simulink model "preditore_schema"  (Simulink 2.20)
settings: Solver=VariableStepDiscrete  StartTime=0.0  StopTime=40.0  RelTol=1e-3  AbsTol=1e-6
libraries: simulink x3

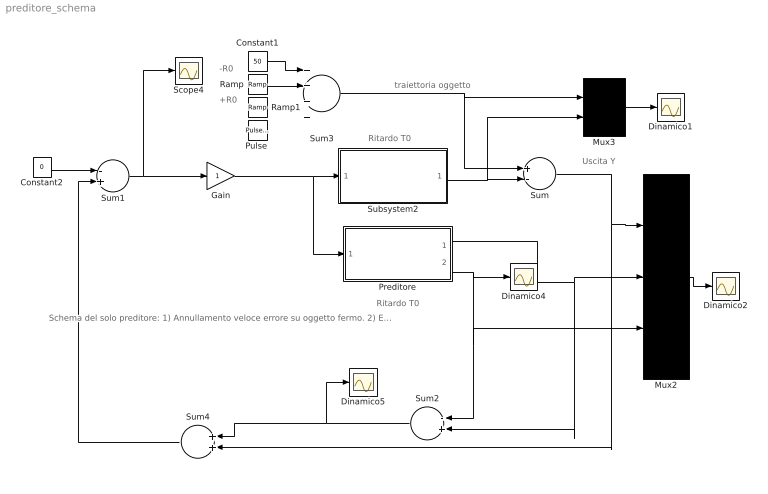
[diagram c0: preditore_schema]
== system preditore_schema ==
  note: traiettoria oggetto
  note: -R0
  note: +R0
  note: Ritardo T0
  note: Ritardo T0
  note: Uscita Y
  note: Schema del solo preditore: 1) Annullamento veloce errore su oggetto fermo. 2) Errore a regime su oggetto in movimento, ma questo sarebbe atteso dato che un proporzionale Kp=1 non e' di per se in grado di annullare l'errore a regime.
  Constant1 : Constant  Value=50
  Constant2 : Constant  Value=0
  Dinamico{1..2,4..5} (4 alike) : Scope
  Gain : Gain  Gain=1
  Mux2 : Mux  Inputs=3
  Mux3 : Mux  Inputs=2
  Preditore : Subsystem  mask(Modello del Puma 260 in Alter Mode){Ts=.260}
      mask prompts: Ts "Tempo di Campionamento Ts della seriale"
      mask help: Questo blocco racchiude il comportamento dinamico del Puma 260 pilotato dalla seriale. La rappresentazione e' a variabili di stato.
      mask init:
      | K=10; % attenuazione del guadagno puma.
      | A=[0,0,0,0,0,0,0,0,0,0;
      | 1,0,0,0,0,0,0,0,0,0;
      | 0,1,0,0,0,0,0,0,0,0;
      | 0,0,1,0,0,0,0,0,0,0;
      | 0,0,0,1,0,0,0,0,0,0;
      | 0,0,0,0,1,0,0,0,0,0;
      | 0,0,0,0,0,1,0,0,0,0;
      | 0,0,0,0,0,0,1,0,0,0;
      | 0,0,0,0,0,0,0,1,0,0;
      | 0,0,0,0,0,0,0,0,1/K,1];
      | B=[1;0;0;0;0;0;0;0;0;0];
      | C=[0,0,0,0,0,0,0,0,0,1;
      | 1/K,1/K,1/K,1/K,1/K,1/K,1/K,1/K,1/K,1];
      | D=[0;0];
  "Pulse " : simulink/Sources/Pulse Generator  period=30  duty=10  amplitude=-50  start=30
  Ramp : simulink/Sources/Ramp  slope=-26  start=10  X0=0
  Ramp1 : simulink/Sources/Ramp  slope=+50  start=25  X0=0
  Scope4 : Scope
  Subsystem2 : Subsystem  mask(Modello del Puma 260 in Alter Mode){Ts=.260}
      mask prompts: Ts "Tempo di Campionamento Ts della seriale"
      mask help: Questo blocco racchiude il comportamento dinamico del Puma 260 pilotato dalla seriale. La rappresentazione e' a variabili di stato.
      mask init:
      | K=10; % attenuazione del guadagno puma.
      | A=[0,0,0,0,0,0,0,0,0,0;
      | 1,0,0,0,0,0,0,0,0,0;
      | 0,1,0,0,0,0,0,0,0,0;
      | 0,0,1,0,0,0,0,0,0,0;
      | 0,0,0,1,0,0,0,0,0,0;
      | 0,0,0,0,1,0,0,0,0,0;
      | 0,0,0,0,0,1,0,0,0,0;
      | 0,0,0,0,0,0,1,0,0,0;
      | 0,0,0,0,0,0,0,1,0,0;
      | 0,0,0,0,0,0,0,0,1/K,1];
      | B=[1;0;0;0;0;0;0;0;0;0];
      | C=[0,0,0,0,0,0,0,0,0,1];
      | D=[0];
  Sum : Sum  Inputs=+-
  Sum1 : Sum  Inputs=-+
  Sum2 : Sum  Orientation=left  Inputs=-+
  Sum3 : Sum  Inputs=++++
  Sum4 : Sum  Orientation=left  Inputs=++
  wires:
  Mux2/1 -> Dinamico2/1
  Subsystem2/1(Out1) -> Sum/2, Mux3/2
  Mux3/1 -> Dinamico1/1
  Constant1/1 -> Sum3/1
  Sum/1 -> Mux2/1, Sum4/2
  Preditore/1(Out1) -> Mux2/2, Sum2/2
  Preditore/2(Out2) -> Dinamico4/1, Sum2/1, Mux2/3
  Sum3/1 -> Mux3/1, Sum/1
  Sum1/1 -> Scope4/1, Gain/1
  Sum4/1 -> Sum1/2
  Constant2/1 -> Sum1/1
  Sum2/1 -> Sum4/1, Dinamico5/1
  Ramp/1 -> Sum3/2
  Gain/1 -> Subsystem2/1(In1), Preditore/1(In1)

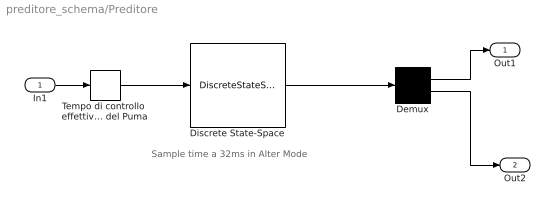
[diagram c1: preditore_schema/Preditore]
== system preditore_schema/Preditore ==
  note: Sample time a 32ms in Alter Mode
  In1 : Inport  Port=1  PortWidth=-1  SampleTime=-1
  Demux : Demux  Outputs=2
  Discrete State-Space : DiscreteStateSpace  A=A  B=B  C=C  D=D  X0=0  SampleTime=.033
  Tempo di controllo  effettivo Ts del Puma : ZeroOrderHold  SampleTime=Ts
  Out1 : Outport  Port=1
  Out2 : Outport  Port=2
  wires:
  In1/1 -> Tempo di controllo  effettivo Ts del Puma/1
  Discrete State-Space/1 -> Demux/1
  Tempo di controllo  effettivo Ts del Puma/1 -> Discrete State-Space/1
  Demux/1 -> Out1/1
  Demux/2 -> Out2/1

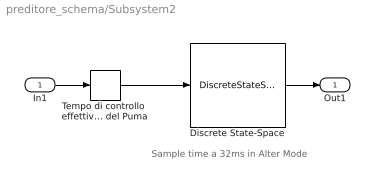
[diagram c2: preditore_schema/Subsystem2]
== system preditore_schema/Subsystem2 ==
  note: Sample time a 32ms in Alter Mode
  In1 : Inport  Port=1  PortWidth=-1  SampleTime=-1
  Discrete State-Space : DiscreteStateSpace  A=A  B=B  C=C  D=D  X0=0  SampleTime=.033
  Tempo di controllo  effettivo Ts del Puma : ZeroOrderHold  SampleTime=Ts
  Out1 : Outport  Port=1
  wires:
  In1/1 -> Tempo di controllo  effettivo Ts del Puma/1
  Discrete State-Space/1 -> Out1/1
  Tempo di controllo  effettivo Ts del Puma/1 -> Discrete State-Space/1
